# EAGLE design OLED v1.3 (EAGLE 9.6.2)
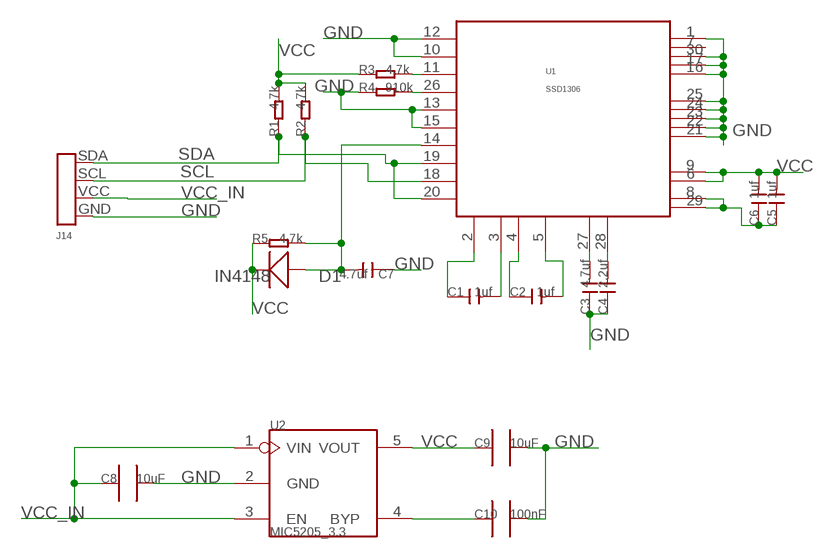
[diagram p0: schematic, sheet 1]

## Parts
C1  1uf  C-0603  [C0603]
C2  1uf  C-0603  [C0603]
C3  4.7uf  C-0603  [C0603]
C4  2.2uf  C-0603  [C0603]
C5  1uf  C-0603  [C0603]
C6  1uf  C-0603  [C0603]
C7  4.7uf  C-0603  [C0603]
C8  10uF  C0805_S  [0805_S]
C9  10uF  C0805_S  [0805_S]
C10  100nF  C0603_S  [0603_S]
D1  IN4148  D'0805'  [SOD323]
J14  OLED1.3  [OLED1.3]
R1  4.7k  R-0603  [R0603]
R2  4.7k  R-0603  [R0603]
R3  4.7k  R-0603  [R0603]
R4  910k  R-0603  [R0603]
R5  4.7k  R-0603  [R0603]
U1  SSD1306  [SSD1306]
U2  MIC5205_3.3  MIC5025_X.X  [SOT23-5]

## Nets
GND: C3.1 C4.1 C7.1 C8.2 C9.2 C10.2 J14.GND R4.1 U1.1(NC_1) U1.10(BS0) U1.12(BS2) U1.13(CS#) U1.15(D/C#) U1.16(R/W#) U1.17(E/RD#) U1.21(D3) U1.22(D4) U1.23(D5) U1.24(D6) U1.25(D7) U1.30(NC_3) U2.2(GND)
N$1: R3.2 U1.11(BS1)
N$2: R4.2 U1.26(IREF)
N$3: C1.2 U1.3(C2N)
N$4: C7.2 D1.+ R5.2 U1.14(RES#)
N$5: C1.1 U1.2(C2P)
N$6: C2.1 U1.4(C1P)
N$7: C2.2 U1.5(C1N)
N$8: C3.2 U1.27(VCOMH)
N$9: C4.2 U1.28(VCC)
N$10: C10.1 U2.4(BYP)
N$11: C5.1 C6.1 U1.8(VSS) U1.29(VLSS)
SCL: J14.SCL R2.1 U1.18(D0)
SDA: J14.SDA R1.1 U1.19(D1) U1.20(D2)
VCC: C5.2 C6.2 C9.1 D1.- R1.2 R2.2 R3.1 R5.1 U1.6(VBAT) U1.9(VDD) U2.5(VOUT)
VCC_IN: C8.1 J14.VCC U2.1(VIN) U2.3(EN)
Unconnected: U1.7(NC_2)

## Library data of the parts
C1-C7 = Discrete:C*: Ceramic Capacitors
C8 C9 = CPT_SMD:C0805
C10 = CPT_SMD:C0603
D1 = Discrete:D*
J14 = smart pump:OLED1.3
R1-R5 = Discrete:R*
U1 = IC:SSD1306
U2 = ICs_v54:MIC5025_X.X

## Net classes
0 default: width 0.203 mm, drill 0.305 mm, clearance 0.203 mm

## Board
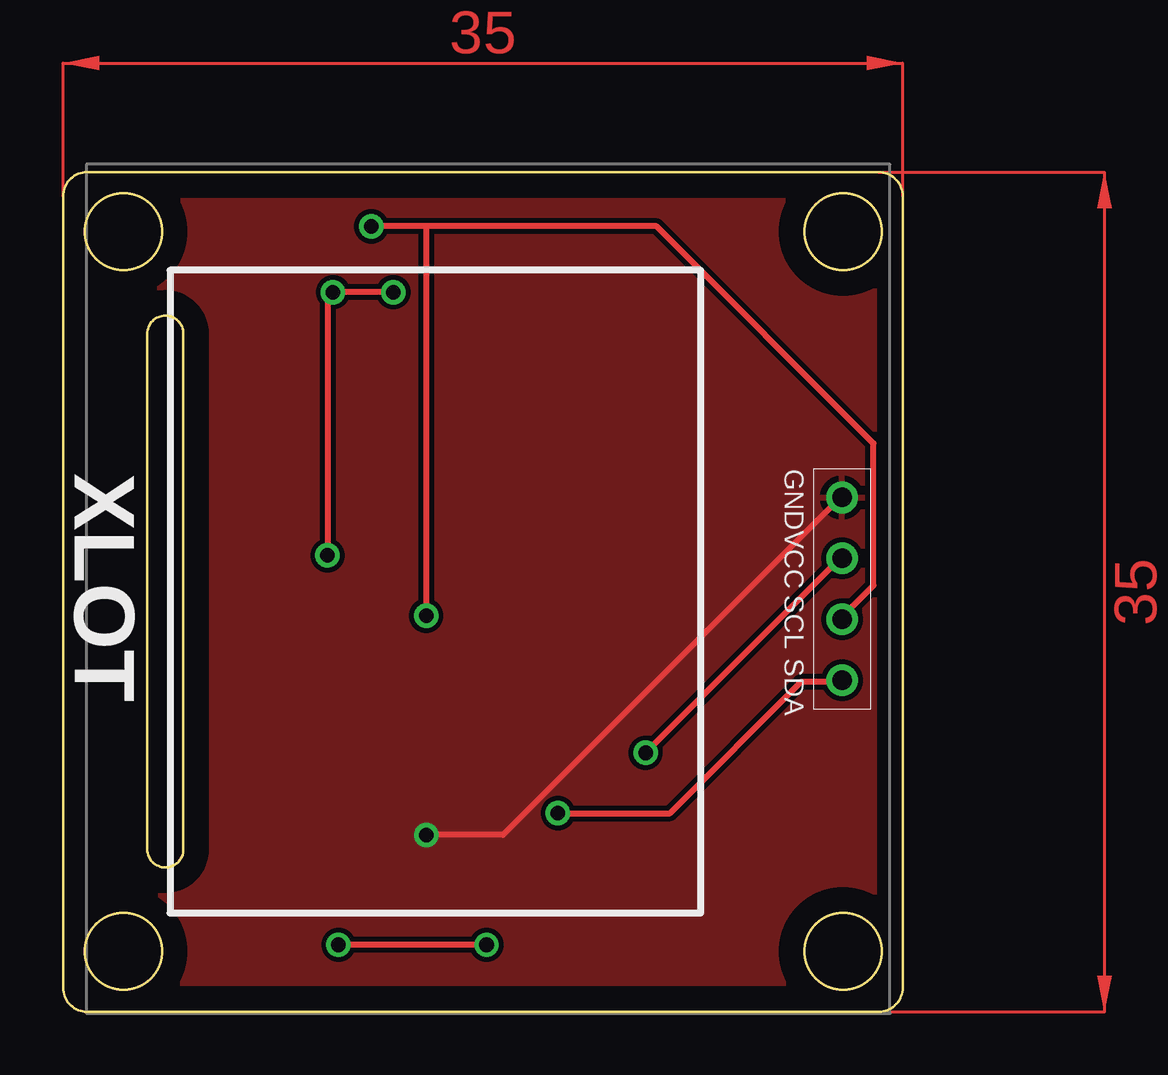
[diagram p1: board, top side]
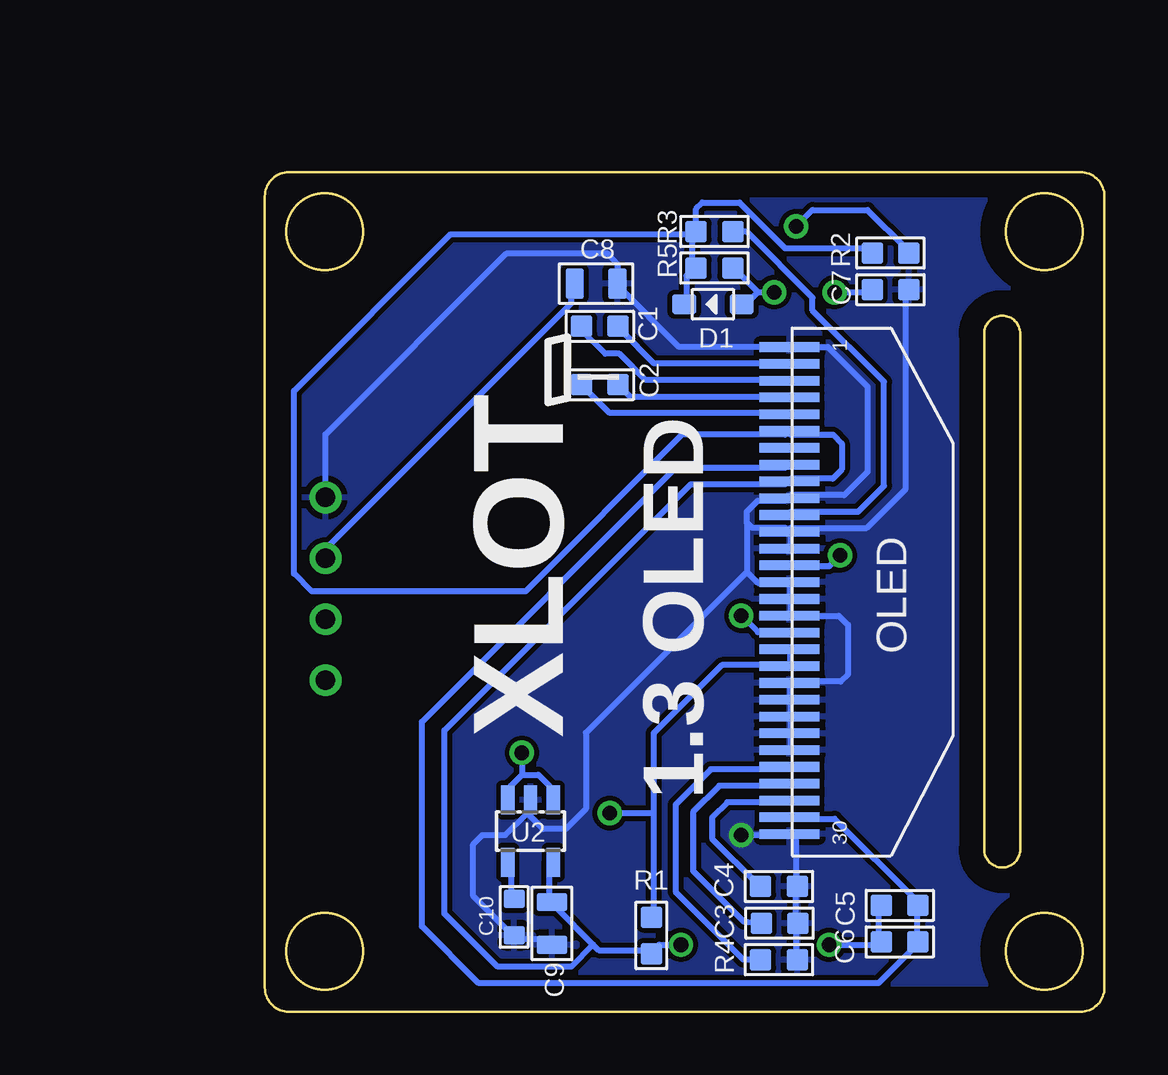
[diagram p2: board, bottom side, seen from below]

Size 35 x 35 mm. Coordinates in mm from the lower left corner, seen from the top.
Outline: 0,34 0,1 arc90 1,0 34,0 arc90 35,1 35,34 arc90 34,35 1,35 arc90 0,34
Outline: 3.51,6.77 3.51,28.27 arc-180 5.01,28.27 5.01,6.77 arc-180 3.51,6.77
Outline: circle at 2.51,2.52 radius 1.6
Outline: circle at 2.51,32.52 radius 1.6
Outline: circle at 32.51,2.52 radius 1.6
Outline: circle at 32.51,32.52 radius 1.6
Copper layers (1*16): Top 0.035mm / dielectric 1.5mm / Bottom 0.035mm
Design rules "default *": minimum track width 10mil, minimum drill 24mil, track to track 8mil, track to pad 8mil, pad to pad 8mil, via to via 8mil, smd to smd 8mil, copper to edge 40mil, drill to drill 8mil, minimum pad ring 10mil, minimum via ring 8mil, stop-mask expansion 4mil, vias tented up to drill 100mil, thermal gap 10mil

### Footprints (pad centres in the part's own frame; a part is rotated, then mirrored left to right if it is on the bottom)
C0603 = smd 0.889 x 0.889: 1 -0.762,0; 2 0.762,0
0805_S = smd 0.762 x 1.27: 1 -0.889,0; 2 0.889,0
0603_S = smd 0.762 x 0.889: 1 -0.762,0; 2 0.762,0
SOD323 = smd 1 x 0.8: + -1.2,0; - 1.2,0
OLED1.3 = drill 0.813: GND -3.89,-0.25; SCL 1.19,-0.25; SDA 3.73,-0.25; VCC -1.35,-0.25
R0603 = smd 0.889 x 0.889: 1 -0.762,0; 2 0.762,0
SSD1306 = smd 0.4 x 2.5: 1 -10.094,-0.115; 2 -9.394,-0.115; 3 -8.694,-0.115; 4 -7.994,-0.115; 5 -7.294,-0.115; 6 -6.594,-0.115; 7 -5.894,-0.115; 8 -5.194,-0.115; 9 -4.494,-0.115; 10 -3.794,-0.115; 11 -3.094,-0.115; 12 -2.394,-0.115; 13 -1.694,-0.115; 14 -0.994,-0.115; 15 -0.294,-0.115; 16 0.406,-0.115; 17 1.106,-0.115; 18 1.806,-0.115; 19 2.506,-0.115; 20 3.206,-0.115; 21 3.906,-0.115; 22 4.606,-0.115; 23 5.306,-0.115; 24 6.006,-0.115; 25 6.706,-0.115; 26 7.406,-0.115; 27 8.106,-0.115; 28 8.806,-0.115; 29 9.506,-0.115; 30 10.206,-0.115
SOT23-5 = smd 0.55 x 1.2: 1 -0.95,-1.3; 2 0,-1.3; 3 0.95,-1.3; 4 0.95,1.3; 5 -0.95,1.3

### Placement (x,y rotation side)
C1  21.03,28.58 180 bottom
C2  21.03,26.15 180 bottom
C3  13.54,3.69 180 bottom
C4  13.57,5.22 180 bottom
C5  8.53,4.43 180 bottom
C6  8.53,2.91 180 bottom
C7  8.92,30.1 180 bottom
C8  21.19,30.35 0 bottom
C9  23.03,3.68 270 bottom
C10  24.6,3.95 270 bottom
D1  16.32,29.49 180 bottom
J14  32.72,17.55 270 top
R1  18.89,3.18 270 bottom
R2  8.92,31.63 180 bottom
R3  16.26,32.53 0 bottom
R4  13.57,2.17 180 bottom
R5  16.26,31 0 bottom
U1  13.01,17.62 270 bottom
U2  23.93,7.53 180 bottom

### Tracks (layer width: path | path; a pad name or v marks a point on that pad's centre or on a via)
GND  (via drill 0.61)
  Top 0.254: v15.14,7.37 18.34,7.37 32.28,21.31 J14.GND
  Bottom 0.254: C9.2 23.14,2.79 23.37,3.02 24.51,3.02 C10.2 24.74,3.25 26.31,4.83 26.31,6.98 25.93,7.37 24.97,7.37 24.05,8.28 | 24.05,8.28 24.05,8.74 U2.2 24.05,8.28 | U1.25 13.08,11.02 13.08,11.48 U1.24 13.08,11.71 13.08,12.17 U1.23 13.08,12.39 13.08,12.85 U1.22 13.08,13.08 13.08,13.54 U1.21 13.08,13.77 11,13.77 10.69,14.07 10.69,16.13 11.07,16.51 13.08,16.51 | 13.08,17.2 13.08,16.51 | 13.08,17.2 13.08,17.88 U1.15 13.31,17.88 14.45,17.88 14.91,18.34 | 13.08,17.2 U1.16 | C7.1 8.28,30 8.28,21.79 9.91,20.17 13.08,20.17 U1.12 | U1.13 13.08,19.48 13.08,19.94 U1.12 | 14.91,20.4 14.91,20.85 14.45,21.31 13.31,21.31 U1.10 13.08,21.54 10.85,21.54 9.88,22.5 9.88,26.06 11.53,27.71 13.08,27.71 U1.1 13.31,27.71 17.73,27.71 20.3,30.29 C8.2 20.3,31.17 20.69,31.6 24.94,31.6 32.47,24.07 J14.GND | 14.91,20.4 14.68,20.17 13.31,20.17 U1.12 | 14.91,20.4 14.91,18.34 | 13.08,16.51 U1.17 | 24.05,8.28 23.39,7.62 22.45,7.62 21.62,8.46 21.62,11.63 14.91,18.34 | R4.1 12.85,2.34 12.85,3.48 C3.1 12.85,3.71 12.85,5.08 C4.1 12.85,5.31 12.85,7.14 13.08,7.37 U1.30 13.31,7.37 v15.14,7.37
  pour Bottom: -0.41,35.28 -0.41,-0.23 35.18,-0.23 35.18,35.18 -0.31,35.18
  pour Top: -0.41,35.33 -0.41,-0.23 35.18,-0.23 35.18,35.18 -0.25,35.18
N$1
  Bottom 0.254: R3.2 15.37,32.51 14.91,32.51 12.17,29.77 12.17,29.24 9.19,26.26 9.19,21.92 10.26,20.85 13.08,20.85 U1.11
N$2
  Bottom 0.254: R4.2 15.05,2.17 17.88,5 17.88,8.64 16.41,10.11 13.31,10.11 U1.26
N$3
  Bottom 0.254: C1.2 21.77,28.4 20.8,27.43 20.22,27.43 19.13,26.34 13.31,26.34 U1.3
N$4  (via drill 0.61)
  Top 0.254: v13.77,30 v11.25,30 11.02,29.77 v11.02,19.02
  Bottom 0.254: v11.25,30 9.88,30 C7.2 | 14.45,30 v13.77,30 | 14.45,30 14.91,29.54 D1.+ | 14.45,30 15.37,30.91 R5.2 | v11.02,19.02 11.48,18.57 13.08,18.57 U1.14
N$5
  Bottom 0.254: C1.1 20.17,28.4 20.14,28.4 18.77,27.03 13.31,27.03 U1.2
N$6
  Bottom 0.254: U1.4 13.31,25.65 19.78,25.65 C2.1
N$7
  Bottom 0.254: C2.2 21.77,26.11 20.62,24.97 13.31,24.97 U1.5
N$8
  Bottom 0.254: C3.2 15.05,3.77 17.14,5.87 17.14,8.33 16.05,9.42 13.31,9.42 U1.27
N$9
  Bottom 0.254: C4.2 14.45,5.31 16.36,7.21 16.36,8.1 15.72,8.74 13.31,8.74 U1.28
N$10
  Bottom 0.254: C10.1 24.74,4.85 24.74,6.22 U2.4
N$11
  Bottom 0.254: U1.29 13.08,8.05 11.25,8.05 7.82,4.62 C5.1 7.82,4.39 7.82,3.02 C6.1 7.82,2.79 9.42,1.19 26.09,1.19 28.45,3.56 28.45,12.09 17.86,22.68 13.31,22.68 U1.8
SCL  (via drill 0.61)
  Top 0.254: 15.14,32.74 24.74,32.74 33.78,23.7 33.78,17.78 32.51,16.51 J14.SCL | 15.14,32.74 v12.85,32.74 | 15.14,32.74 v15.14,16.51
  Bottom 0.254: v12.85,32.74 12.17,33.43 9.88,33.43 8.28,31.83 R2.1 | v15.14,16.51 14.45,15.82 13.31,15.82 U1.18
SDA  (via drill 0.61)
  Top 0.254: v20.62,8.28 25.3,8.28 30.78,13.77 32.28,13.77 J14.SDA
  Bottom 0.254: 18.8,8.28 18.8,11.61 15.95,14.45 13.31,14.45 U1.20 13.08,14.45 13.08,15.14 U1.19 | 18.8,8.28 18.8,4.17 R1.1 | 18.8,8.28 v20.62,8.28
VCC  (via drill 0.61)
  Top 0.254: v17.65,2.79 v11.48,2.79
  Bottom 0.254: R2.2 9.88,31.83 13.31,31.83 15.21,33.73 16.76,33.73 17.02,33.48 R3.1 17.2,32.51 17.2,32.41 | 17.2,32.41 17.2,31.14 R5.1 17.2,30.91 17.42,30.68 17.42,29.54 D1.- | C5.2 9.42,4.39 9.42,3.02 C6.2 9.42,2.79 v11.48,2.79 | 21.31,2.79 22.91,4.39 C9.1 23.14,4.62 23.14,6.22 U2.5 | 21.31,2.79 21.08,2.57 19.02,2.57 R1.2 18.8,2.57 18.57,2.79 v17.65,2.79 | 21.31,2.79 22.22,1.88 25.3,1.88 27.51,4.09 27.51,11.73 17.25,22 13.31,22 U1.9 13.08,22.22 11.33,22.22 10.95,22.61 10.95,23.7 11.3,24.05 13.08,24.05 U1.6 13.31,24.05 17.6,24.05 24.13,17.53 33.05,17.53 33.78,18.26 33.78,25.88 27.25,32.41 17.2,32.41
VCC_IN  (via drill 0.61)
  Top 0.254: v24.28,10.79 32.28,18.8 J14.VCC
  Bottom 0.254: 24.28,9.88 23.6,9.88 23.14,9.42 23.14,8.97 U2.1 | 24.28,9.88 24.74,9.42 24.74,8.97 U2.3 | C8.1 22.22,30.23 22.22,29.54 32.28,19.48 32.28,19.02 J14.VCC | v24.28,10.79 24.28,9.88
(copper drawn outside any net)
  shapes: Top area x2

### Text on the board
tPlace: GND | XLOT | VCC | SCL | SDA
bPlace: I | XLOT | 1.3 OLED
